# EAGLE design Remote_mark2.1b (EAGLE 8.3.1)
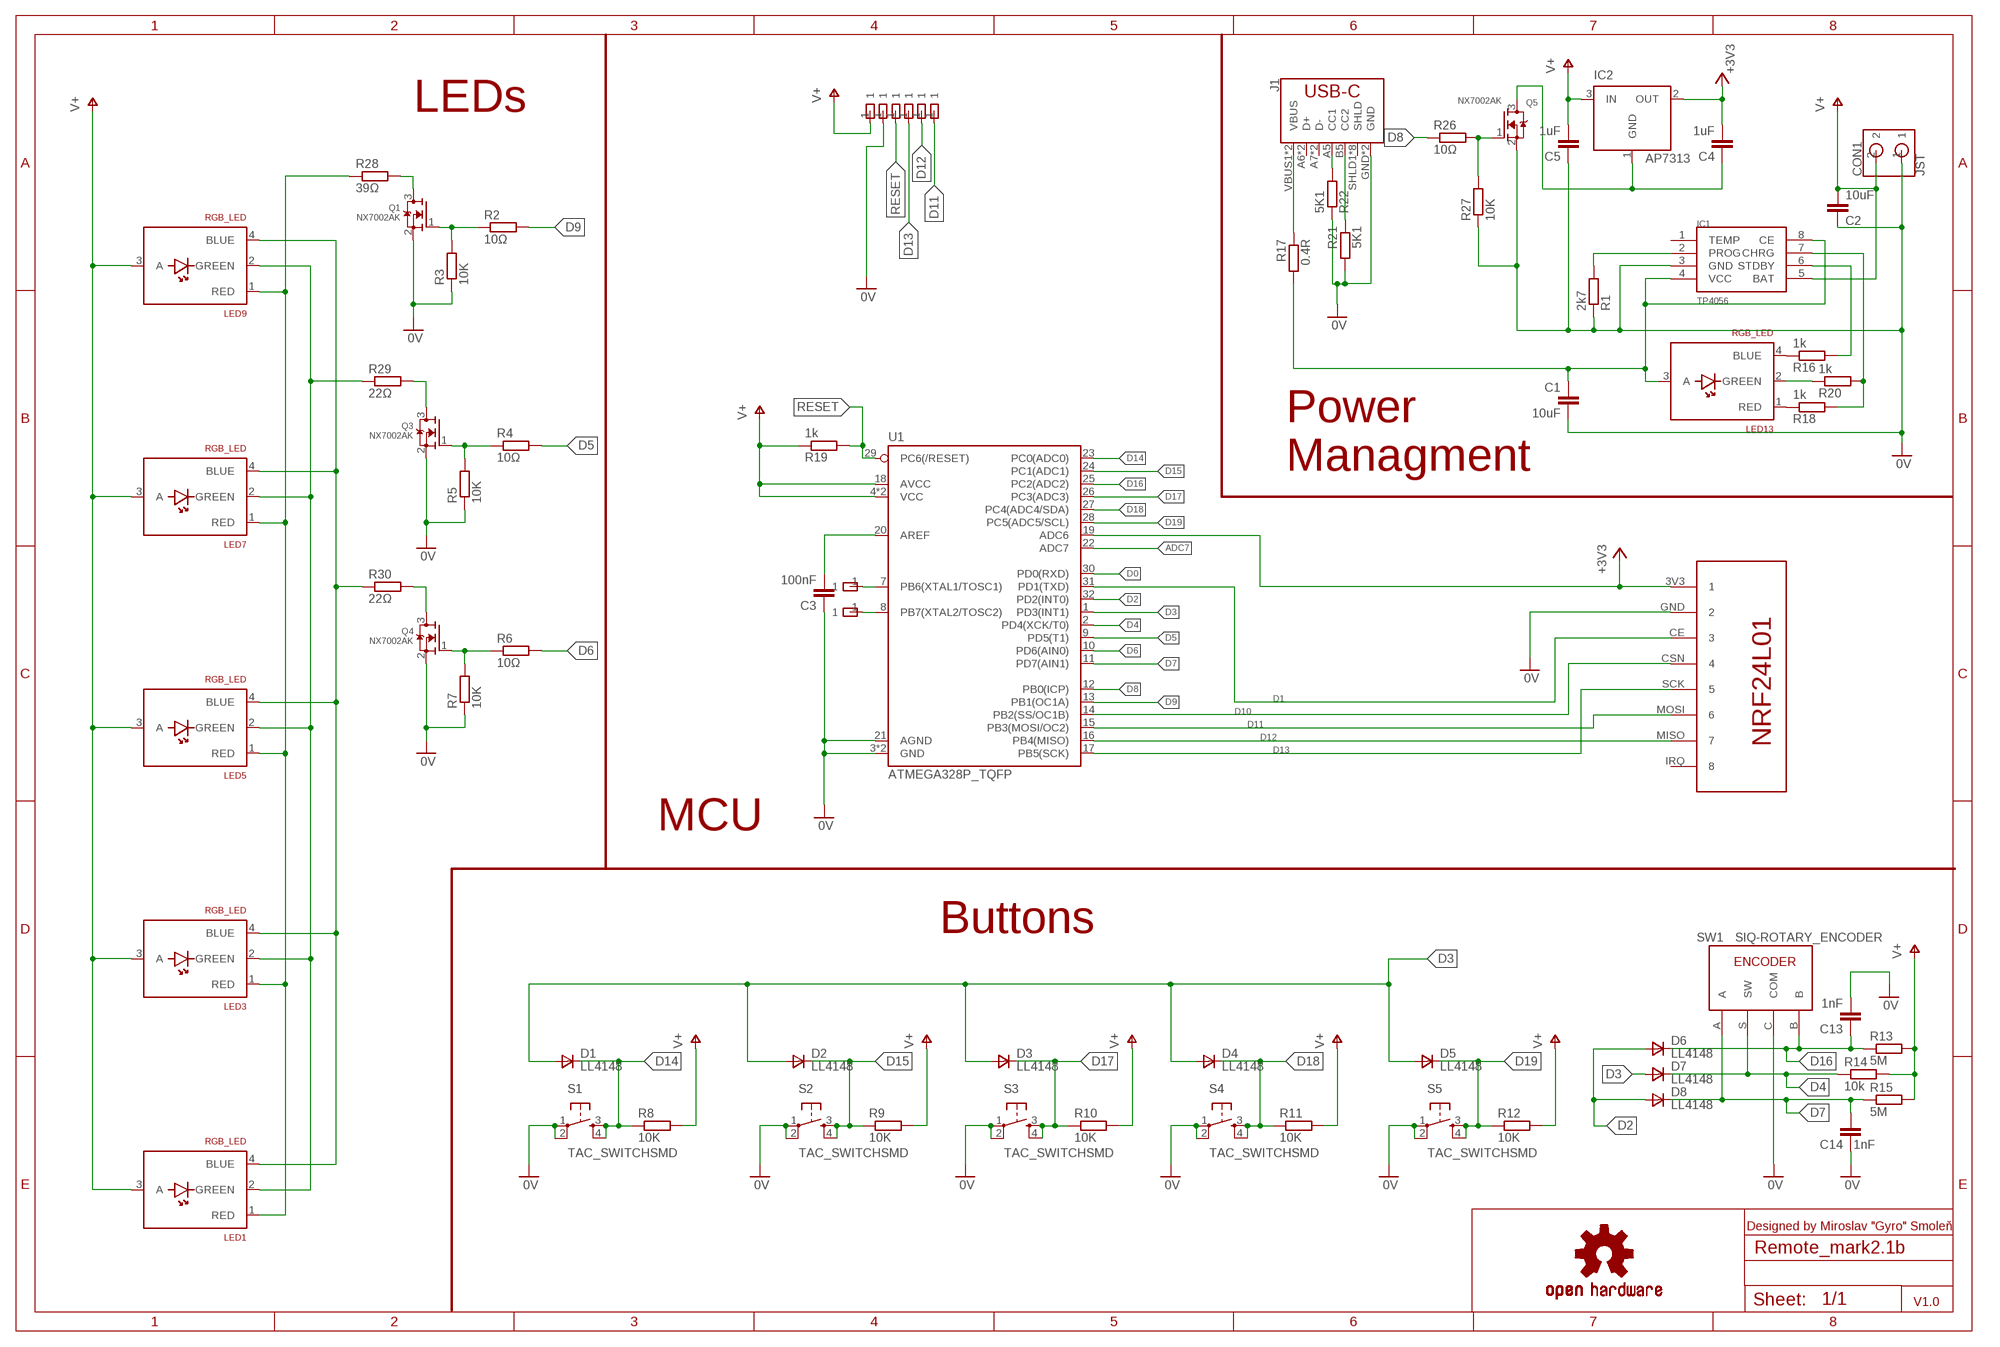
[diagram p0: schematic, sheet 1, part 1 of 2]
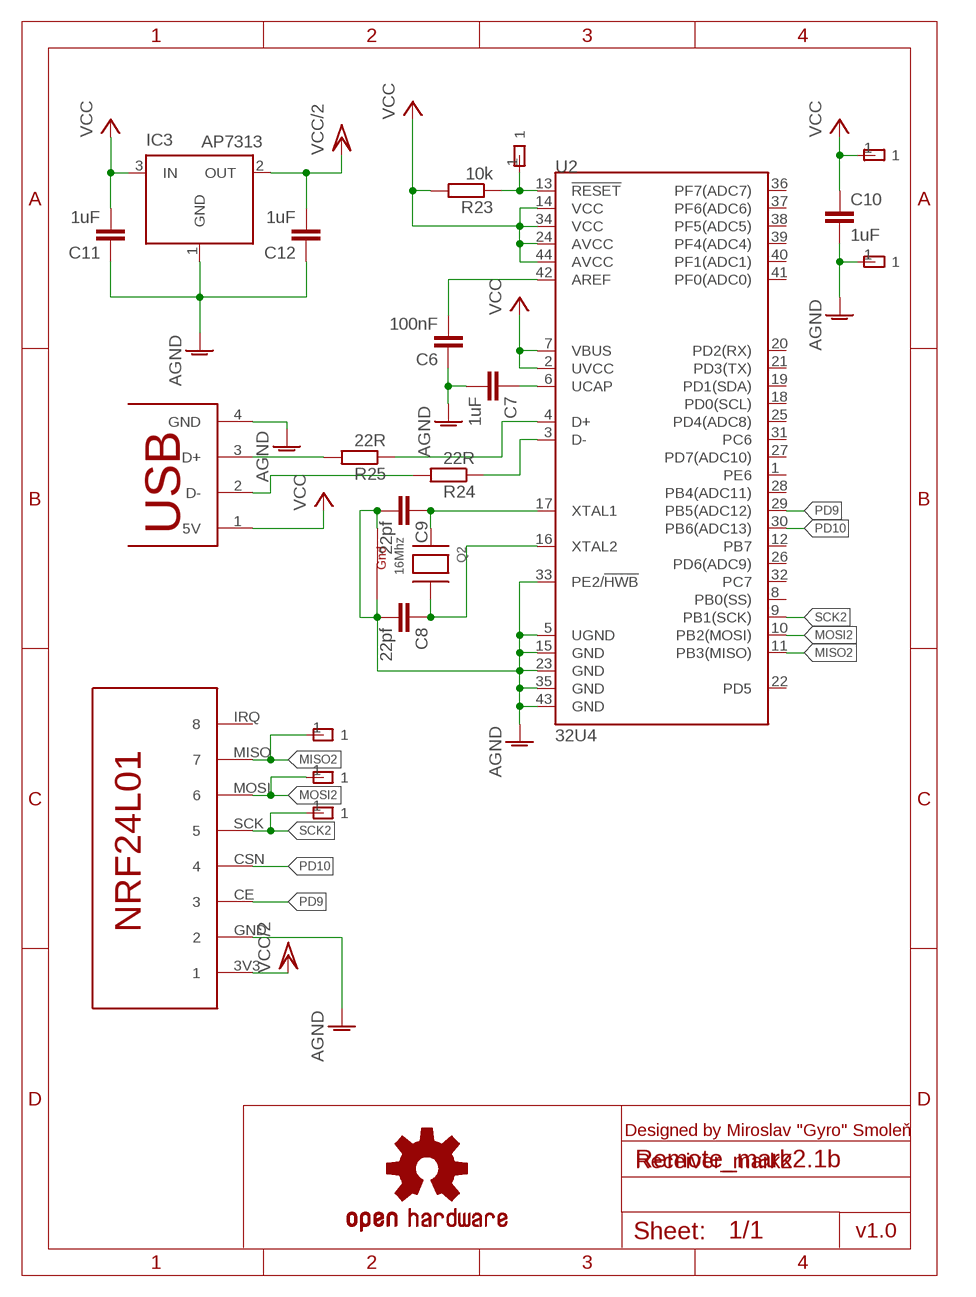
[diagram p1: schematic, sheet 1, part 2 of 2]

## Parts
C1  10uF  C-EUC0805  [C0805]
C2  10uF  C-EUC0805  [C0805]
C3  100nF  C-EUC0603  [C0603]
C4  1uF  C-EUC0603  [C0603]
C5  1uF  C-EUC0603  [C0603]
C6  100nF  C-EUC0603  [C0603]
C7  1uF  C-EUC0603  [C0603]
C8  22pf  C-EUC0603  [C0603]
C9  22pf  C-EUC0603  [C0603]
C10  1uF  C-EUC0603  [C0603]
C11  1uF  C-EUC0603  [C0603]
C12  1uF  C-EUC0603  [C0603]
C13  1nF  C-EUC0603  [C0603]
C14  1nF  C-EUC0603  [C0603]
CON1  JST  JST_PH2.0_BAT_CON  [JST_PH_2.0_2PIN_CONNECTOR]
D1  LL4148  DSOD323  [SOD323]
D2  LL4148  DSOD323  [SOD323]
D3  LL4148  DSOD323  [SOD323]
D4  LL4148  DSOD323  [SOD323]
D5  LL4148  DSOD323  [SOD323]
D6  LL4148  DSOD323  [SOD323]
D7  LL4148  DSOD323  [SOD323]
D8  LL4148  DSOD323  [SOD323]
IC1  TP4056  [SOP-8]
IC2  AP7313  AP7313_LINEAR_PWR_REG  [SOT23R]
IC3  AP7313  AP7313_LINEAR_PWR_REG  [SOT23R]
J1  USB_C16PIN  [USB-C-16P]
LED1  RGB_LED  [1.6X1.6_RGB_LED]
LED3  RGB_LED  [1.6X1.6_RGB_LED]
LED5  RGB_LED  [1.6X1.6_RGB_LED]
LED7  RGB_LED  [1.6X1.6_RGB_LED]
LED9  RGB_LED  [1.6X1.6_RGB_LED]
LED13  RGB_LED  [1.6X1.6_RGB_LED]
LOGO1  OSHW-LOGOS  [OSHW-LOGO-S]
LOGO2  OSHW-LOGOS  [OSHW-LOGO-S]
Q1  NX7002AK  MOSFET-NREFLOW  [SOT23]
Q2  16Mhz  XTAL-4-3225  [NX3225]
Q3  NX7002AK  MOSFET-NREFLOW  [SOT23]
Q4  NX7002AK  MOSFET-NREFLOW  [SOT23]
Q5  NX7002AK  MOSFET-NREFLOW  [SOT23]
R1  2k7  R-EU_R0603  [R0603]
R2  10Ω  R-EU_R0603  [R0603]
R3  10K  R-EU_R0603  [R0603]
R4  10Ω  R-EU_R0603  [R0603]
R5  10K  R-EU_R0603  [R0603]
R6  10Ω  R-EU_R0603  [R0603]
R7  10K  R-EU_R0603  [R0603]
R8  10K  R-EU_R0603  [R0603]
R9  10K  R-EU_R0603  [R0603]
R10  10K  R-EU_R0603  [R0603]
R11  10K  R-EU_R0603  [R0603]
R12  10K  R-EU_R0603  [R0603]
R13  5M  R-EU_R0603  [R0603]
R14  10k  R-EU_R0603  [R0603]
R15  5M  R-EU_R0603  [R0603]
R16  1k  R-EU_R0603  [R0603]
R17  0.4R  R-EU_R0805  [R0805]
R18  1k  R-EU_R0603  [R0603]
R19  1k  R-EU_R0603  [R0603]
R20  1k  R-EU_R0603  [R0603]
R21  5K1  R-EU_R0603  [R0603]
R22  5K1  R-EU_R0603  [R0603]
R23  10k  R-EU_R0603  [R0603]
R24  22R  R-EU_R0603  [R0603]
R25  22R  R-EU_R0603  [R0603]
R26  10Ω  R-EU_R0603  [R0603]
R27  10K  R-EU_R0603  [R0603]
R28  39Ω  R-EU_R0603  [R0603]
R29  22Ω  R-EU_R0603  [R0603]
R30  22Ω  R-EU_R0603  [R0603]
S1  TAC_SWITCHSMD  [TACTILE-SWITCH-SMD]
S2  TAC_SWITCHSMD  [TACTILE-SWITCH-SMD]
S3  TAC_SWITCHSMD  [TACTILE-SWITCH-SMD]
S4  TAC_SWITCHSMD  [TACTILE-SWITCH-SMD]
S5  TAC_SWITCHSMD  [TACTILE-SWITCH-SMD]
SW1  SIQ-ROTARY_ENCODER  [SIQ-02FVS3]
U1  ATMEGA328P_TQFP  [TQFP32-08]
U2  32U4  ATMEGA32U4TQFP-44  [TQFP44]
U$1  NRF24  [NRF24L01_SMT]
U$2  PAD_POGO_PIN  [POGO_PAD]
U$3  PAD_POGO_PIN  [POGO_PAD]
U$4  PAD_POGO_PIN  [POGO_PAD]
U$5  PAD_POGO_PIN  [POGO_PAD]
U$6  PAD_POGO_PIN  [POGO_PAD]
U$7  PAD_POGO_PIN  [POGO_PAD]
U$8  USB-A  [USB-A-SMT-MALE]
U$9  NRF24  [NRF24L01_SMT]
U$10  PAD_POGO_PIN  [POGO_PAD]
U$11  PAD_POGO_PIN  [POGO_PAD]
U$12  PAD_POGO_PIN  [POGO_PAD]
U$13  PAD_POGO_PIN  [POGO_PAD]
U$14  PAD_POGO_PIN  [POGO_PAD]
U$15  PAD_POGO_PIN  [POGO_PAD]
U$16  PAD_POGO_PIN  [POGO_PAD]
U$17  PAD_POGO_PIN  [POGO_PAD]

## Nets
0V: C1.2 C2.1 C3.1 C5.1 C13.2 C14.1 CON1.1 IC1.3(GND) J1.GND J1.GND2(GND) Q1.2(S) Q3.2(S) Q4.2(S) Q5.2(S) R1.1 R3.1 R5.1 R7.1 R21.2 R22.1 R27.1 S1.1 S1.2 S2.1 S2.2 S3.1 S3.2 S4.1 S4.2 S5.1 S5.2 SW1.C(COM) U1.3(GND) U1.5(GND) U1.21(AGND) U$1.GND U$3.1
+3V3: C4.2 IC2.2(OUT) U1.19(ADC6) U$1.3V3
ADC7: U1.22(ADC7)
AGND: C6.1 C7.2 C8.2 C9.2 C10.2 C11.1 C12.1 IC3.1(GND) Q2.2(G2) Q2.4(G1) U2.5(UGND) U2.15(GND) U2.23(GND) U2.33(PE2/!HWB) U2.35(GND) U2.43(GND) U$8.4(GND) U$9.GND U$17.1
D0: U1.30(PD0(RXD))
D1: U1.31(PD1(TXD)) U$1.CE
D2: D6.2(A) D8.2(A) U1.32(PD2(INT0))
D3: D1.2(A) D2.2(A) D3.2(A) D4.2(A) D5.2(A) D7.2(A) U1.1(PD3(INT1))
D4: D7.1(C) R14.1 SW1.S(SW) U1.2(PD4(XCK/T0))
D5: R4.2 U1.9(PD5(T1))
D6: R6.2 U1.10(PD6(AIN0))
D7: C14.2 D8.1(C) R15.1 SW1.A U1.11(PD7(AIN1))
D8: R26.1 U1.12(PB0(ICP))
D9: R2.2 U1.13(PB1(OC1A))
D10: U1.14(PB2(SS/OC1B)) U$1.CSN
D11: U1.15(PB3(MOSI/OC2)) U$1.MOSI U$7.1
D12: U1.16(PB4(MISO)) U$1.MISO U$6.1
D13: U1.17(PB5(SCK)) U$1.SCK U$5.1
D14: D1.1(C) R8.1 S1.3 S1.4 U1.23(PC0(ADC0))
D15: D2.1(C) R9.1 S2.3 S2.4 U1.24(PC1(ADC1))
D16: C13.1 D6.1(C) R13.1 SW1.B U1.25(PC2(ADC2))
D17: D3.1(C) R10.1 S3.3 S3.4 U1.26(PC3(ADC3))
D18: D4.1(C) R11.1 S4.3 S4.4 U1.27(PC4(ADC4/SDA))
D19: D5.1(C) R12.1 S5.3 S5.4 U1.28(PC5(ADC5/SCL))
MISO2: U2.11(PB3(MISO)) U$9.MISO U$12.1
MOSI2: U2.10(PB2(MOSI)) U$9.MOSI U$13.1
N$1: IC1.2(PROG) R1.2
N$2: LED1.1(RED) LED3.1(RED) LED5.1(RED) LED7.1(RED) LED9.1(RED) R28.1
N$3: C1.1 IC1.4(VCC) IC1.8(CE) LED13.3(A) R17.2
N$4: LED1.2(GREEN) LED3.2(GREEN) LED5.2(GREEN) LED7.2(GREEN) LED9.2(GREEN) R29.1
N$5: Q1.1(G) R2.1 R3.2
N$6: Q3.1(G) R4.1 R5.2
N$7: LED1.4(BLUE) LED3.4(BLUE) LED5.4(BLUE) LED7.4(BLUE) LED9.4(BLUE) R30.1
N$8: Q4.1(G) R6.1 R7.2
N$9: IC1.6(STDBY) R16.2
N$10: IC1.7(CHRG) R18.2 R20.2
N$11: LED13.4(BLUE) R16.1
N$12: LED13.1(RED) R18.1
N$13: C9.1 Q2.1(X1) U2.17(XTAL1)
N$14: C3.2 U1.20(AREF)
N$16: LED13.2(GREEN) R20.1
N$17: J1.B5(CC2) R21.1
N$18: J1.A5(CC1) R22.2
N$19: C8.1 Q2.3(X2) U2.16(XTAL2)
N$20: C6.2 U2.42(AREF)
N$21: J1.VBUS1(VBUS) J1.VBUS2(VBUS) R17.1
N$22: U1.7(PB6(XTAL1/TOSC1)) U$10.1
N$23: C7.1 U2.6(UCAP)
N$24: R23.1 U2.13(!RESET) U$15.1
N$25: U1.8(PB7(XTAL2/TOSC2)) U$11.1
N$26: R24.1 U2.3(D-)
N$27: R25.1 U2.4(D+)
N$28: R25.2 U$8.3(D+)
N$29: R24.2 U$8.2(D-)
N$30: Q5.1(G) R26.2 R27.2
N$31: C4.1 IC2.1(GND) Q5.3(D)
N$32: Q1.3(D) R28.2
N$33: Q3.3(D) R29.2
N$34: Q4.3(D) R30.2
PD9: U2.29(PB5(ADC12)) U$9.CE
PD10: U2.30(PB6(ADC13)) U$9.CSN
RESET: R19.2 U1.29(PC6(/RESET)) U$4.1
SCK2: U2.9(PB1(SCK)) U$9.SCK U$14.1
V+: C2.2 C5.2 CON1.2 IC1.5(BAT) IC2.3(IN) LED1.3(A) LED3.3(A) LED5.3(A) LED7.3(A) LED9.3(A) R8.2 R9.2 R10.2 R11.2 R12.2 R13.2 R14.2 R15.2 R19.1 U1.4(VCC) U1.6(VCC) U1.18(AVCC) U$2.1
VCC: C10.1 C11.2 IC3.3(IN) R23.2 U2.2(UVCC) U2.7(VBUS) U2.14(VCC) U2.24(AVCC) U2.34(VCC) U2.44(AVCC) U$8.1(5V) U$16.1
VCC/2: C12.2 IC3.2(OUT) U$9.3V3
Unconnected: IC1.1(TEMP) J1.A6(D+) J1.A7(D-) J1.B6(D+) J1.B7(D-) J1.SHLD1(SHLD) J1.SHLD2(SHLD) J1.SHLD3(SHLD) J1.SHLD4(SHLD) J1.SHLD5(SHLD) J1.SHLD6(SHLD) J1.SHLD7(SHLD) J1.SHLD8(SHLD) U2.1(PE6) U2.8(PB0(SS)) U2.12(PB7) U2.18(PD0(SCL)) U2.19(PD1(SDA)) U2.20(PD2(RX)) U2.21(PD3(TX)) U2.22(PD5) U2.25(PD4(ADC8)) U2.26(PD6(ADC9)) U2.27(PD7(ADC10)) U2.28(PB4(ADC11)) U2.31(PC6) U2.32(PC7) U2.36(PF7(ADC7)) U2.37(PF6(ADC6)) U2.38(PF5(ADC5)) U2.39(PF4(ADC4)) U2.40(PF1(ADC1)) U2.41(PF0(ADC0)) U$1.IRQ U$9.IRQ

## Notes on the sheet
- LEDs
- Power
  Managment
- MCU
- Buttons
- Designed by Miroslav "Gyro" Smoleň | Designed by Miroslav "Gyro" Smoleň
- Receiver_mark2
- V1.0 | v1.0

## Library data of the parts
C1-C14 = rcl:C-EU: CAPACITOR, European symbol
CON1 = Gyro_library:JST_PH2.0_BAT_CON
D1-D8 = zetex:D: DIODE; MPN: CDSOD323-T05C; OC_FARNELL: 1824860; OC_NEWARK: 79R6078
IC1 = TP4056:TP4056
IC2 IC3 = Gyro_library:AP7313_LINEAR_PWR_REG: 1.2V Voltage Reference 50ppm/°C, SOT23, 3-Terminal Source: Data sheet; MF: MAXIM; MPN: MAX6520EUR-T; OC_FARNELL: unknown; OC_NEWARK: 02J4586
J1 = SparkFun-Connectors:USB_C: USB Type C 16Pin Connector Super Speed pins not available on the 16-pin purely SMD connector so this part is best for USB 2.0 implementations. D1 and D2 are tied together enabling D+/- no matter which way the cable is plugged into the connector. The two channel configuration pins (CC1/2) are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; PROD_ID: CONN-14122
LED1 LED3 LED5 LED7 LED9 LED13 = Gyro_library:RGB_LED
LOGO1 LOGO2 = SparkFun-Aesthetics:OSHW-LOGO: Open-Source Hardware (OSHW) Logo
Q1 Q3-Q5 = adafruit:MOSFET-N: N-Channel Mosfet 2N7002E - 60V 260mA SOT23 [Digikey: 2N7002ET1GOSTR-ND] - REEL BSH103 - 30V 850mA SOT23 [Digikey: 568-5013-1-ND]
Q2 = adafruit:XTAL-4: Classic 4-pin 3.2 x 2.5mm crystal
R1-R30 = rcl:R-EU_: RESISTOR, European symbol
S1-S5 = SparkFun-Retired:TAC_SWITCH: Momentary Switch Button commonly used for reset or general input. Spark Fun Electronics SKU : COM-00097 SMT- SWCH-08247; PROD_ID: SWCH-08247
SW1 = Gyro_library:SIQ-ROTARY_ENCODER
U1 = SparkFun-IC-Microcontroller:ATMEGA328P_TQFP: Popular 328P in QFP Storefront component: ATmega328 - TQFP (COM-13448) Datasheet SparkFun Products SparkFun RedBoard - Programmed with Arduino (DEV-12757) Arduino Pro Mini 328 - 5V/16MHz (DEV-11113) Arduino Pro Mini 328 - 3.3V/8MHz (DEV-11114) SparkFun OpenLog (DEV-13712) SparkFun MicroView - OLED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; PROD_ID: IC-09069
U2 = SparkFun-IC-Microcontroller:ATMEGA32U4: Atmel MCU, 32KByte Atmel 44-pin 8-bit Microcontroller with 32KBytes of ISP Flash and USB Controller Datasheet SparkFun Products LilyPad Arduino USB - ATmega32U4 Board (DEV-12049) Pro Micro - 5V/16MHz (DEV-12640) Pro Micro - 3.3V/8MHz (DEV-12587) Fio v3 - ATmega32U4 (DEV-11520) Qduino Mini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; PROD_ID: IC-11161
U$1 U$9 = Gyro_library:NRF24: SMD version of NRF24L01 wireless transceiver module. Made by Gyro: https://www.youtube.com/c/gyro1
U$2-U$7 U$10-U$17 = Gyro_library:PAD_POGO_PIN
U$8 = Gyro_library:USB-A

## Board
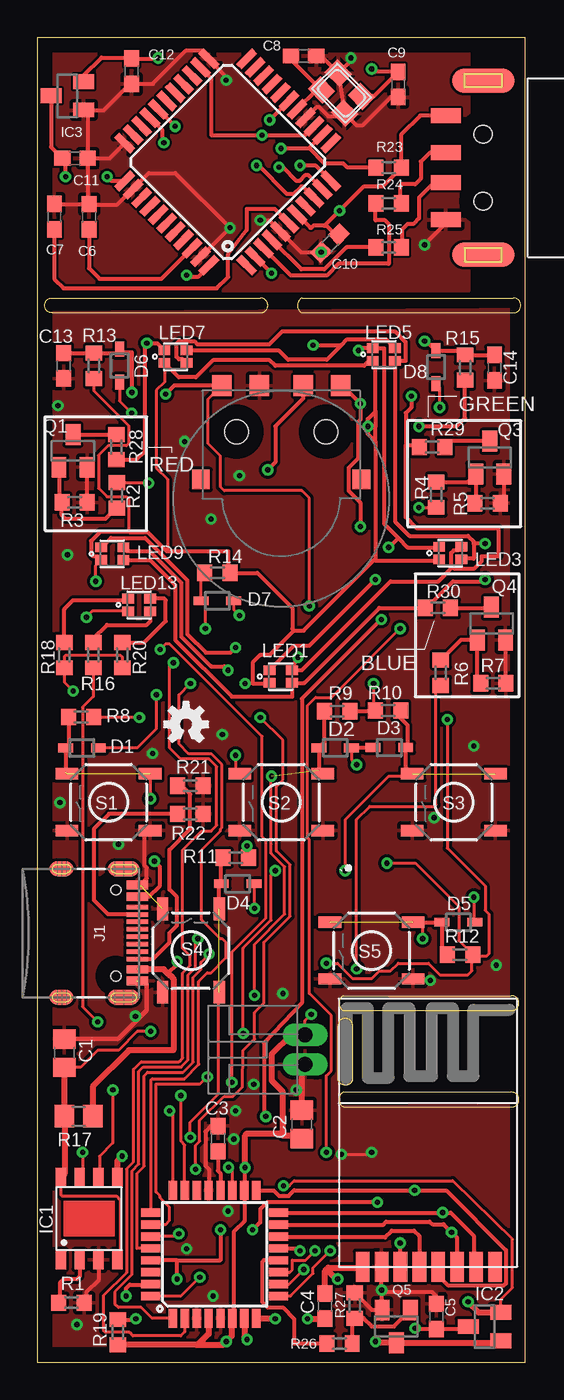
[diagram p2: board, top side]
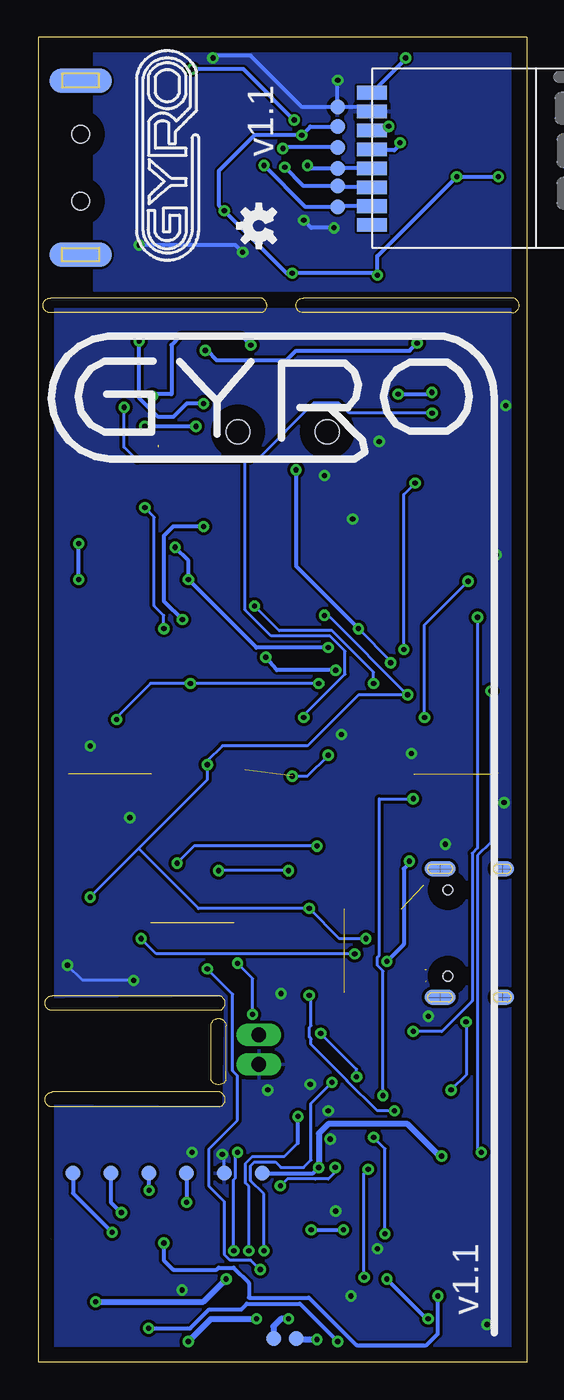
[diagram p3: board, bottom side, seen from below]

Size 32.8 x 89 mm. Coordinates in mm from the lower left corner, seen from the top.
Outline: 0,0 32.8,0 32.8,89 0,89 0,0
Copper layers (1*16): Top 0.035mm / dielectric 1.5mm / Bottom 0.035mm
Design rules "default": minimum track width 6mil, minimum drill 0.35mm, track to track 6mil, track to pad 6mil, pad to pad 6mil, via to via 6mil, smd to smd 6mil, copper to edge 40mil, drill to drill 6mil, minimum pad ring 10mil, minimum via ring 8mil, stop-mask expansion 4mil, vias tented up to drill 0mil, thermal gap 10mil
Milling: 20 lines

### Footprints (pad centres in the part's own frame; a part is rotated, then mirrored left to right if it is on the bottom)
C0805 = smd 1.3 x 1.5: 1 -0.95,0; 2 0.95,0
C0603 = smd 1.1 x 1: 1 -0.85,0; 2 0.85,0
JST_PH_2.0_2PIN_CONNECTOR = drill 1 long: 1 -1,0; 2 1,0
SOD323 = smd 1 x 0.6: 1 -1.1,0; 2 1.1,0
SOP-8 = smd 1.3 x 0.7: 1 -2.75,1.905; 2 -2.75,0.635; 3 -2.75,-0.635; 4 -2.75,-1.905; 5 2.75,-1.905; 6 2.75,-0.635; 7 2.75,0.635; 8 2.75,1.905
SOT23R = smd 1 x 1.4: 1 -0.95,-1.1; 2 0.95,-1.1; 3 0,1.1
USB-C-16P = smd 0.3 x 1.45: A5 -1.25,0; A6 -0.25,0; A7 0.25,0; A8 1.25,0; B5 1.75,0; B6 0.75,0; B7 -0.75,0; B8 -1.75,0 | smd 0.6 x 1.45: GND -3.225,0; GND2 3.225,0 | smd 1 x 2.1: SHLD1 -4.32,-0.915; SHLD2 4.32,-0.915 | smd 1 x 2.1 bottom: SHLD3 -4.32,-0.915; SHLD4 4.32,-0.915 | smd 1 x 1.6: SHLD5 -4.32,-5.095; SHLD8 4.32,-5.095 | smd 1 x 1.6 bottom: SHLD6 -4.32,-5.095; SHLD7 4.32,-5.095 | smd 0.55 x 1.45: VBUS1 -2.45,0; VBUS2 2.45,0 | hole 0.65: -2.89,-1.445; 2.89,-1.445
1.6X1.6_RGB_LED = smd 0.8 x 0.65: 1 -0.75,0.425; 2 0.75,0.425; 3 -0.75,-0.425; 4 0.75,-0.425
SOT23 = smd 1 x 1.4: 1 -0.95,-1.1; 2 0.95,-1.1; 3 0,1.1
NX3225 = smd 1.4 x 1.2: 1 -1.1,-0.8; 2 1.1,-0.8; 3 1.1,0.8; 4 -1.1,0.8
R0603 = smd 1 x 1.1: 1 -0.85,0; 2 0.85,0
R0805 = smd 1.3 x 1.5: 1 -0.95,0; 2 0.95,0
TACTILE-SWITCH-SMD = smd 1.524 x 0.762: 1 -2.794,1.905; 2 2.794,1.905; 3 -2.794,-1.905; 4 2.794,-1.905
SIQ-02FVS3 = smd 1.3 x 1.4: A -4,-7.6; B 4,-7.6; C 1.475,-7.6; S -1.475,-7.6 | smd 1.2 x 1.3: P$5 5.4,-1.3; P$6 -5.4,-1.3 | hole 1.6: -3,-4.5; 3,-4.5
TQFP32-08 = smd 1.27 x 0.559: 1 -4.293,2.8; 2 -4.293,2; 3 -4.293,1.2; 4 -4.293,0.4; 5 -4.293,-0.4; 6 -4.293,-1.2; 7 -4.293,-2; 8 -4.293,-2.8; 17 4.293,-2.8; 18 4.293,-2; 19 4.293,-1.2; 20 4.293,-0.4; 21 4.293,0.4; 22 4.293,1.2; 23 4.293,2; 24 4.293,2.8 | smd 0.559 x 1.27: 9 -2.8,-4.293; 10 -2,-4.293; 11 -1.2,-4.293; 12 -0.4,-4.293; 13 0.4,-4.293; 14 1.2,-4.293; 15 2,-4.293; 16 2.8,-4.293; 25 2.8,4.293; 26 2,4.293; 27 1.2,4.293; 28 0.4,4.293; 29 -0.4,4.293; 30 -1.2,4.293; 31 -2,4.293; 32 -2.8,4.293
TQFP44 = smd 1.5 x 0.5: 1 -5.8,4; 2 -5.8,3.2; 3 -5.8,2.4; 4 -5.8,1.6; 5 -5.8,0.8; 6 -5.8,0; 7 -5.8,-0.8; 8 -5.8,-1.6; 9 -5.8,-2.4; 10 -5.8,-3.2; 11 -5.8,-4; 23 5.8,-4; 24 5.8,-3.2; 25 5.8,-2.4; 26 5.8,-1.6; 27 5.8,-0.8; 28 5.8,0; 29 5.8,0.8; 30 5.8,1.6; 31 5.8,2.4; 32 5.8,3.2; 33 5.8,4 | smd 0.5 x 1.5: 12 -4,-5.8; 13 -3.2,-5.8; 14 -2.4,-5.8; 15 -1.6,-5.8; 16 -0.8,-5.8; 17 0,-5.8; 18 0.8,-5.8; 19 1.6,-5.8; 20 2.4,-5.8; 21 3.2,-5.8; 22 4,-5.8; 34 4,5.8; 35 3.2,5.8; 36 2.4,5.8; 37 1.6,5.8; 38 0.8,5.8; 39 0,5.8; 40 -0.8,5.8; 41 -1.6,5.8; 42 -2.4,5.8; 43 -3.2,5.8; 44 -4,5.8
NRF24L01_SMT = smd 2 x 0.914: 3V3 -9,4.4; CE -9,1.86; CSN -9,0.59; GND -9,3.13; IRQ -9,-4.49; MISO -9,-3.22; MOSI -9,-1.95; SCK -9,-0.68
POGO_PAD = smd 1 x 1: 1 0,0
USB-A-SMT-MALE = smd 1 x 2: 1 3.5,2.5; 2 1,2.5; 3 -1,2.5; 4 -3.5,2.5 | smd 1.651 x 4.191 bottom: P$1 -5.842,0; P$2 5.842,0 | smd 1.651 x 4.191: P$3 5.842,0; P$5 -5.842,0 | hole 1.2: 2.25,0; -2.25,0

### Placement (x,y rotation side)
C1  1.83,20.76 90 top
C2  17.78,15.98 270 top
C3  12.15,15.02 270 top
C4  19.35,3.78 90 top
C5  26.82,3.08 270 top
C6  3.48,76.94 270 top
C7  1.16,76.94 90 top
C8  17.91,87.74 0 top
C9  24.26,85.83 270 top
C10  19.68,75.16 225 top
C11  2.54,80.87 180 top
C12  6.35,86.71 90 top
C13  1.78,66.93 270 top
C14  30.73,66.8 90 top
CON1  18,21 90 top
D1  3.01,41.26 0 top
D2  20.03,41.27 0 top
D3  23.66,41.29 180 top
D4  13.47,32.15 0 top
D5  28.3,29.56 0 top
D6  5.53,66.94 270 top
D7  12.1,51.15 0 top
D8  26.8,66.84 270 top
IC1  3.49,9.65 90 top
IC2  30.06,2.4 90 top
IC3  2.03,85.06 90 top
J1  6.73,28.83 270 top
LED1  16.36,46.06 0 top
LED3  27.76,54.35 0 top
LED5  23.29,67.69 0 top
LED7  9.3,67.55 0 top
LED9  5.04,54.31 0 top
LED13  6.85,50.87 0 top
LOGO1  10,42.85 0 top
LOGO2  18,76.33 90 bottom
Q1  2.41,61.21 0 top
Q2  20.45,85.24 135 top
Q3  30.41,60.76 0 top
Q4  30.52,49.62 0 top
Q5  24.13,2.41 180 top
R1  2.3,4 180 top
R2  5.34,58.23 90 top
R3  2.52,57.75 180 top
R4  26.81,58.27 270 top
R5  30.27,57.7 180 top
R6  27.12,46.32 270 top
R7  30.65,45.6 180 top
R8  2.95,43.34 0 top
R9  20.16,43.73 0 top
R10  23.59,43.78 180 top
R11  13.35,33.89 0 top
R12  28.41,27.39 0 top
R13  3.81,66.93 270 top
R14  12.11,53.02 0 top
R15  28.74,66.81 270 top
R16  3.77,47.5 270 top
R17  2.79,16.53 180 top
R18  1.82,47.5 270 top
R19  5.43,2.02 90 top
R20  5.71,47.5 270 top
R21  10.29,38.73 0 top
R22  10.29,36.83 180 top
R23  23.62,80.24 0 top
R24  23.62,77.82 0 top
R25  23.62,74.89 0 top
R26  20.32,1.27 0 top
R27  21.34,3.81 270 top
R28  5.33,61.47 90 top
R29  26.54,61.47 0 top
R30  26.92,50.67 0 top
S1  4.8,37.62 180 top
S2  16.4,37.62 180 top
S3  28,37.62 180 top
S4  10.33,27.65 90 top
S5  22.47,27.65 180 top
SW1  16.4,58 180 top
U1  11.92,7.25 90 top
U2  12.81,80.62 135 top
U$1  26.27,15.42 90 top
U$2  17.78,12.7 270 bottom
U$3  20.32,12.7 270 bottom
U$4  22.86,12.7 270 bottom
U$5  25.4,12.7 270 bottom
U$6  27.94,12.7 270 bottom
U$7  30.48,12.7 270 bottom
U$8  29.97,80.24 90 top
U$9  1.4,80.87 0 bottom
U$10  15.5,1.6 0 bottom
U$11  17,1.6 0 bottom
U$12  12.7,77.6 0 bottom
U$13  12.7,79 0 bottom
U$14  12.7,80.18 0 bottom
U$15  12.7,81.6 0 bottom
U$16  12.7,83 0 bottom
U$17  12.7,84.3 0 bottom

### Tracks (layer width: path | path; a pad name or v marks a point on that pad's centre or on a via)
0V  (via drill 0.35)  (2 unrouted)
  Top 0.203: S5.1 26.32,25.75 v26.42,25.65 | v20.45,13.97 22.35,13.97 v22.48,14.1
  Top 0.254: R27.1 22.48,3.51 Q5.2 23.14,3.55 23.14,4.71 | 23.14,4.71 U$1.GND | R3.1 3.37,60.11 Q1.2 | Q3.2 31.36,57.95 R5.1 | Q4.2 31.47,45.63 R7.1 | IC1.3 4.12,5.52 3.3,4.7 3.3,4.15 R1.1 | J1.GND 6.91,32.05 7.37,32.51 7.37,33.23 7.22,33.38 7.22,35.33 S1.1 | C3.1 11.68,15.87 11.3,15.49 11.3,13.21 11.56,12.95 11.56,11.58 U1.21 | C5.1 26.82,4.43 26.54,4.7 23.15,4.7 23.14,4.71
  Top 0.305: C1.2 5.46,21.71 7.37,23.62 7.37,25.4 7.24,25.53 6.81,25.53 6.78,25.56
  Top 0.406: C2.1 17.78,19.78 CON1.1
  Bottom 0.203: v26.42,25.65 29.84,25.65 v30.86,26.67 | U$3.1 20.32,13.84 v20.45,13.97
  other vias: 11.68,56.64 9.91,61.85 13.59,59.56 1.4,64.26 5.46,34.8 7.75,40.89 12.45,42.16 29.34,41.4 11.81,4.45 2.67,2.54 23.15,4.85 13.21,14.99 16.51,24.77 17.4,18.29 26.67,36.58 1.52,37.59 6.6,23.24 12.83,10.16 2.03,54.23 10.03,7.62 13.34,16.89 14.55,18.66
  pour Top (isolate 0.2): 0,-0.13 33.53,-0.13 34.16,17.27 20.32,17.14 20.19,24.64 34.04,24.51 34.67,70.74 0,70.48
  pour Bottom (isolate 0.2): -0.51,-0.64 33.91,-0.64 33.53,17.27 20.32,17.14 20.19,24.64 34.67,24.51 33.91,70.74 -0.51,70.74
+3V3  (via drill 0.35)  (1 unrouted)
  Top 0.203: IC2.2 31.16,4.24 31.94,5.01 31.94,8.25 | U1.19 13.12,12.83 v12.86,13.09 | v16.55,11.85 16.93,11.85 17.27,12.19 27.92,12.19 31.95,8.26
  Top 0.406: C4.2 19.35,6.14 19.45,6.24 | 19.45,6.24 19.56,6.35 21.8,6.35 U$1.3V3 | IC2.2 29.67,3.35 v28.96,4.06 | v20.19,5.59 20.1,5.59 19.45,6.24
  Bottom 0.203: v12.86,13.09 12.86,12.79 13.34,12.32 14.19,12.32 | 14.19,12.32 | v16.55,11.85 16.08,12.32 14.19,12.32
  Bottom 0.406: v28.96,4.06 21.72,4.06 v20.19,5.59
AGND  (via drill 0.35)
  Top 0.254: C10.2 17.74,74.56 U2.5 15.58,76.71 v14.99,76.71 | Q2.2 Q2.4 | C9.2 23.76,84.97 21.84,83.06 21.5,83.06 Q2.4 | C8.2 19.08,87.74 Q2.2 | C11.1 3.39,83.86 3.22,84.03 | 3.22,84.03 IC3.1 | 3.22,84.03 3.27,84.07 4.45,84.07 6.24,85.86 C12.1 7.76,85.86 10.01,88.11 11.05,88.11 11.56,87.63 11.53,87.53 12.7,86.36 v12.7,86.11 | C11.1 3.39,77.88 C6.1 | C7.2 C6.1 | C6.1 3.54,77.72 5.33,77.72 6.39,78.78 U2.35 6.44,78.83 7.49,79.88 9.27,79.88 v12.95,76.2 11.01,74.25 U2.43 | C11.1 4.86,80.87 U2.33 | U$8.4 27.47,76.49 v26.04,75.06 | U2.15 18.06,83.59 18.8,84.33 18.92,84.33 19.56,83.69 20.47,83.69 Q2.4 | v21.08,87.61 21.08,87.43 Q2.2
  Bottom 0.254: U$17.1 10.7,84.3 U$9.GND | U$17.1 v12.7,86.11 | v26.04,75.06 19.59,75.06 C10.2 | v12.95,76.2 14.48,76.2 v14.99,76.71 | U$17.1 15.09,84.3 18.54,87.76 20.93,87.76 v21.08,87.61
  other vias: 19.08,74.56
  pour Top: 0,72 29,72 29,89 0,89.13
  pour Bottom: 0,72 29,72 29,89 0,89.13
D1  (via drill 0.35)
  Top 0.254: U$1.CE 24.41,7.97 v24.38,8 | v5.97,4.45 5.97,4.95 6.22,5.21 7.58,5.21 U1.31
  Bottom 0.254: v24.38,8 24.38,6.86 23.75,6.22 20.83,6.22 20.7,6.35 19.68,6.35 18.67,5.33 18.67,4.34 14.63,4.34 11.43,1.14 6.73,1.14 5.97,1.91 v5.97,4.45
D2  (via drill 0.35)
  Top 0.203: D6.2 5.53,64.57 v6.35,63.75 | v27.05,64.14 27.05,65.49 D8.2 | U1.32 9.66,4.45 v10.92,5.71 | v10.64,12.95 10.64,14.58 10.92,14.85 10.92,16.26 12.57,17.86 13.16,17.86 13.79,18.49 13.84,20.95 14.61,21.72 14.61,23.5 15.24,24.13 15.24,28.21 16.99,29.96 16.99,33.43 16.08,34.34 16.08,38.68 16.51,39.12 16.51,41.78 v14.99,43.31
  Bottom 0.203: v6.35,63.75 11.94,63.75 12.61,64.42 14.32,64.42 18.03,60.71 18.48,60.71 18.61,60.58 18.93,60.58 | 18.93,60.58 26.16,60.58 27.05,61.47 v27.05,64.14 | v10.92,5.71 10.92,12.68 v10.64,12.95 | v14.99,43.31 14.99,43.43 12.2,46.22 12.2,47.76 13.23,48.79 17.18,48.79 18.92,50.54 18.92,60.57 18.93,60.58
D3  (via drill 0.35)
  Top 0.203: U1.1 7.71,2.96 6.99,3.68 5.46,3.68 5.21,3.94 5.21,4.73 6.36,5.88 6.36,12.84 6.83,13.31 6.83,19.54 7.13,19.84 9.67,19.84 10.13,20.3 10.13,26.02 10.64,26.52 10.64,28.3 v10.79,28.45 | v14.61,30.48 14.61,32.11 D4.2 | D7.2 13.2,50.55 v13.59,50.16 | v8,44.83 8,42.55 6.73,41.27 4.13,41.27 D1.2 | D2.2 21.13,40.47 v21.46,40.13 | v29.34,31.24 29.34,29.62 D5.2
  Top 0.254: D2.2 22.55,41.27 D3.2
  Bottom 0.203: v10.79,28.45 12.57,28.45 v14.61,30.48 22.05,30.48 26.07,34.5 | v13.59,50.16 13.34,50.16 v8,44.83 11.3,44.83 14.73,41.4 20.45,41.4 21.46,40.39 v21.46,40.13 21.46,39.12 26.07,34.5 | 26.07,34.5 v29.34,31.24
D4  (via drill 0.35)
  Top 0.203: U1.2 9.92,2.05 9.65,1.78 6.42,1.78 6.2,2 4.6,2 4.45,2.16 4.45,4.47 6,6.03 6,12.98 6.48,13.46 6.48,19.68 6.99,20.19 9.53,20.19 9.78,20.45 9.78,26.16 10.29,26.67 10.29,27.3 9.78,27.81 9.78,34.42 11.05,35.69 11.68,35.69 12.06,36.07 12.06,40.01 11.56,40.51 9.65,40.51 8.89,41.27 8.89,46.74 v9.14,46.99 | v11.3,49.28 11.3,50.85 D7.1 11,52.77 R14.1
  Top 0.254: SW1.S 17.88,64.74 16,62.87 16,60.45 v15.49,59.94
  Bottom 0.203: v9.14,46.99 9.14,47.12 v11.3,49.28
  Bottom 0.254: v15.49,59.94 15.49,53.47 v11.3,49.28
D5  (via drill 0.35)
  Top 0.203: v19.68,7.49 18.54,6.35 18.54,5.96 17.03,4.45 U1.9 | v19.43,14.1 19.43,19.25 19.76,19.58 19.76,23.29 18.29,24.77 18.29,35.12 18.18,35.23 18.18,44.12 18.71,44.66 19.76,44.66 v24.38,49.28 | v25.65,57.4 26.79,57.4 R4.2
  Bottom 0.203: v19.68,7.49 19.68,12.27 19.57,12.39 19.57,13.96 v19.43,14.1 | v24.38,49.28 24.38,50.16 25.02,50.8 25.02,56.77 v25.65,57.4
D6  (via drill 0.35)
  Top 0.203: U1.10 16.93,5.25 v17.91,6.22 | v21.46,26.42 21.46,36.45 22.35,37.34 26.67,37.34 26.8,37.47 26.8,45.14 R6.2
  Bottom 0.203: v17.91,6.22 18.55,6.86 19.95,6.86 20.32,7.23 20.32,10.79 21.34,11.81 21.34,14.35 19.43,16.26 19.43,19.25 19.76,19.58 19.76,24.71 v21.46,26.42
D7  (via drill 0.35)
  Top 0.203: U1.11 16.97,6.05 17.14,6.22 17.14,6.86 18.03,6.86 v18.67,7.49
  Top 0.254: C14.2 30.72,67.66 R15.1 28.47,67.94 D8.1 26.16,68.58 v26.04,68.58 | SW1.A 20.51,65.6 v21.72,64.39 21.72,63.29 21.57,63.14 21.57,60.71 20.92,60.07 20.92,58.53 21.72,57.74 v21.72,56.13 | v23.13,49.89 23.09,49.89 17.78,44.58 17.78,24.13 15.24,21.46 15.24,16.76 v15.37,16.51
  Bottom 0.203: 15.37,14.73 16.28,13.82 18.43,13.82 18.9,13.36 18.9,12.04 18.67,11.82 v18.67,7.49
  Bottom 0.254: v21.72,64.39 22.86,64.39 23.75,63.5 24.77,63.5 26.04,64.77 v26.04,68.58 | v21.72,56.13 23.75,56.13 24.38,55.5 24.38,51.14 v23.13,49.89 | 15.37,14.73 v15.37,16.51
D8
  Top 0.254: U1.12 15.23,6.85 15.11,6.73 15.11,4.06 15.49,3.68 16.51,3.68 17.27,2.92 17.27,1.27 R26.1
D9  (via drill 0.35)
  Top 0.203: v13.08,18.8 13.08,27.56 15.37,29.84 15.37,35.05 15.11,35.31 15.11,42.04 8.89,48.26 8.64,48.26 v8.26,47.88 | v7.49,59.05 5.37,59.05 R2.2
  Top 0.254: U1.13 17.5,7.65 v17.65,7.49
  Bottom 0.203: v17.65,7.49 17.65,11.3 18.54,12.19 18.54,13.21 18.29,13.46 16.89,13.46 16.51,13.08 14.99,13.08 14.48,13.59 14.48,17.4 v13.08,18.8 | v8.26,47.88 8.26,58.29 v7.49,59.05
D10
  Top 0.254: U1.14 16.28,8.38 23.37,8.38 23.83,8.84 25.32,8.84 25.68,8.48 U$1.CSN
D11  (via drill 0.35)
  Top 0.254: U$1.MOSI 28.19,6.45 28.19,8.38 v27.85,8.72 27.3,9.27 26.54,9.27 26.36,9.45 23.45,9.45 23.25,9.25 U1.15
  Bottom 0.254: U$7.1 30.48,11.35 v27.85,8.72
D12  (via drill 0.35)
  Top 0.254: U1.16 v27.24,10.05 27.8,10.05 29.34,8.51 29.34,6.57 U$1.MISO
  Bottom 0.254: U$6.1 27.94,10.75 v27.24,10.05
D13  (via drill 0.35)
  Top 0.254: U1.17 15.89,11.54 16.26,11.18 16.89,11.18 17.27,11.56 v25.37,11.54 27.49,11.54 31.5,7.54 31.5,5.3 31.33,5.14 27.65,5.14 26.95,5.84 U$1.SCK
  Bottom 0.254: U$5.1 25.4,11.57 v25.37,11.54
D14  (via drill 0.35)  (2 unrouted)
  Top 0.203: U1.23 9.92,14.59 9.65,14.85 v9.65,17.9 v9.65,17.91 | v7.62,37.85 7.62,39.49 S1.3
  Top 0.254: R8.1 2.1,41.45 D1.1 1.91,39.62
  Bottom 0.203: v9.65,17.91 9.65,26.28 10.03,26.66 10.03,27.19 9.91,27.31 9.91,37.85 v7.62,37.85
D15  (via drill 0.35)  (1 unrouted)
  Top 0.203: U1.24 9.12,16.66 v8.89,16.89 | v14.61,24.64 14.61,28.08 16.63,30.11 16.63,33.28 15.72,34.19 15.72,34.8 15.72,39.34 v15.75,39.37 | v13.34,40.77 13.34,39.79 S2.4
  Top 0.254: S2.3 18.93,39.79 D2.1 19.31,41.66 R9.1
  Bottom 0.203: v8.89,16.89 10.04,16.89 12.06,18.91 12.06,18.92 14.48,21.34 14.48,21.72 14.61,21.84 14.61,22.48 14.48,22.61 14.48,24.51 v14.61,24.64 | v15.75,39.37 14.73,39.37 v13.34,40.77
D16  (via drill 0.35)
  Top 0.203: U1.25 7.63,18.93 7.75,19.05 9.89,19.05 10.85,20 10.85,20.07 10.85,25.58 11.43,26.16 11.68,26.16 12.7,27.18 12.7,28.19 12.45,28.45 12.32,28.45 11.05,29.72 11.05,34.42 12.32,35.69 12.32,35.82 12.42,35.92 12.42,40.15 11.7,40.87 11.43,40.87 10.19,40.87 9.53,41.53 9.53,44.83 v10.29,45.59 | v18.29,50.8 18.29,58.04 17.78,58.55 12.57,58.55 12.32,58.8 12.32,60.87 11.48,61.71 11.48,64.68 SW1.B
  Top 0.254: C13.1 R13.1 5.28,67.78 5.46,67.97 | 5.46,67.97 D6.1 | SW1.B 9.21,65.6 v8.64,65.02 | v6.37,65.15 6.37,67.8 6.35,67.82 5.61,67.82 5.46,67.97
  Bottom 0.203: v10.29,45.59 10.29,46.35 13.08,49.15 16.64,49.15 v18.29,50.8
  Bottom 0.254: v8.64,65.02 6.49,65.02 v6.37,65.15
D17  (via drill 0.35)  (1 unrouted)
  Top 0.203: U1.26 8.62,9.25 8.89,9.53 8.89,10.41 8.26,11.05 8.26,11.18 7.98,11.45 7.98,18.69 10.94,18.69 v11.43,19.18 | v13.84,22.1 13.84,27.82 15.72,29.7 15.72,32.74 v16,33.02 | v20.7,33.02 20.7,36.45 23.62,39.37 25.05,39.37 S3.4
  Top 0.254: S3.4 24.76,39.97 D3.1 24.89,41.42 24.89,42.8 24.44,43.25 R10.1
  Bottom 0.203: v11.43,19.18 11.43,19.68 v13.84,22.1 | v16,33.02 v20.7,33.02
D18  (via drill 0.35)  (1 unrouted)
  Top 0.203: U1.27 9.34,8.45 v9.53,8.64 | v10.29,15.11 10.29,16.13 12.19,18.03 12.19,24.81 S4.3
  Top 0.254: S4.4 12.24,32.01 D4.1 12.37,33.76 R11.1
  Bottom 0.203: v9.53,8.64 9.53,14.35 v10.29,15.11
D19  (via drill 0.35)  (1 unrouted)
  Top 0.203: U1.28 6.71,7.65 6.71,12.69 7.19,13.17 7.19,19.25 7.42,19.48 9.82,19.48 10.49,20.15 10.49,25.87 11,26.38 11,26.87 v11.56,27.43 | v25.91,28.45 25.91,29.24 25.59,29.56
  Top 0.254: S5.3 25.59,29.56 D5.1 27.2,27.75 R12.1
  Bottom 0.203: v11.56,27.43 24.89,27.43 v25.91,28.45
MISO2  (via drill 0.35)
  Top 0.254: v17.65,80.39 18.69,80.39 U2.11
  Bottom 0.254: v17.65,80.39 14.86,77.6 U$12.1 12.65,77.65 U$9.MISO
MOSI2  (via drill 0.35)
  Top 0.254: v16.26,80.26 16.51,80.26 17.4,79.38 17.65,79.38 18.03,79.76 18.19,79.76 U2.10
  Bottom 0.254: v16.26,80.26 14.99,79 U$13.1 12.62,78.92 U$9.MOSI
N$1
  Top 0.254: IC1.2 2.85,5.78 2.67,5.59 1.78,5.59 1.52,5.33 1.52,4.07 R1.2
N$2  (via drill 0.35)
  Top 0.254: v21.59,67.97 21.74,68.11 LED5.1 23.3,68.11 23.3,56.33 24.26,55.37 | LED7.1 8.07,68.45 v7.37,68.45 7.24,68.33 7.24,61.21 6.64,60.62 R28.1 | 24.26,55.37 24.89,54.74 26.97,54.74 LED3.1 | LED1.1 15.62,46.49 17.27,48.13 18.29,48.13 v22.73,52.58 | v23.62,54.74 23.63,54.74 24.26,55.37 | 4.29,54.84 LED9.1 4.31,54.73 4.95,55.37 7.25,55.37 10.08,52.53 10.08,48.91 11.34,47.66 12.99,47.66 v13.34,48.01
  Bottom 0.254: v21.59,67.97 21.49,67.97 20.83,67.31 16.13,67.31 15.49,67.94 7.87,67.94 v7.37,68.45 | v23.62,54.74 22.73,53.85 v22.73,52.58 18.16,48.01 v13.34,48.01
N$3  (via drill 0.35)
  Top 0.203: LED13.3 3.71,50.45 v3.3,50.04 | v7.62,22.23 6.73,22.23 5.46,20.95 4.06,20.95 2.92,19.81 C1.1 | IC1.8 1.58,11.24 1.65,11.18 5.33,11.18 5.59,10.92 5.59,7.09 IC1.4
  Top 0.406: C1.1 1.83,16.54 R17.2 1.84,12.66 IC1.8
  Bottom 0.203: v3.3,50.04 3.3,34.54 3.66,34.18 3.66,24.28 5.71,22.23 v7.62,22.23
N$4  (via drill 0.35)  (1 unrouted)
  Top 0.254: LED5.2 23.44,68.72 20.83,68.72 20.44,68.33 | 20.44,68.33 20.35,68.24 20.35,68.23 19.46,67.33 16.87,67.33 16.26,67.94 10.07,67.94 LED7.2 | 27.91,53.4 27.83,53.48 27.83,54.36 27.99,54.53 28.26,54.53 LED3.2 | 27.91,53.4 27.99,53.32 29.38,53.32 29.87,53.81 29.87,54.14 31.01,54.14 31.01,55.98 29.46,56.01 25.53,56.01 24.77,56.77 24.77,61.59 25.57,61.59 R29.1 | 24.77,61.47 24.77,63.75 25.15,64.14 v25.15,64.9 | v18.54,68.33 20.44,68.33 | 17.26,46.49 LED1.2 | 17.26,46.49 17.78,46.49 23.75,52.45 26.95,52.45 27.91,53.4 | LED9.2 6.04,54.48 7.56,54.48 9.68,52.37 9.68,48.74 11.68,46.74 12.57,46.74 v12.83,46.48 | v17.53,47.35 17.27,46.88 17.26,46.49
  Bottom 0.254: v18.54,68.33 19.18,68.96 23.24,68.96 23.88,68.33 23.88,65.02 25.02,65.02 v25.15,64.9 | v12.83,46.48 16.79,46.48 v17.53,47.35
N$5
  Top 0.254: Q1.1 1.46,57.96 R3.2 1.65,57.73 1.65,56.9 1.91,56.64 4.57,56.64 5.31,57.38 R2.1
N$6
  Top 0.254: R5.2 29.46,57.74 Q3.1 28.93,59.12 R4.1
N$7  (via drill 0.35)
  Top 0.254: LED7.4 9.8,67.37 9.53,67.37 9.37,67.53 9.37,68.42 9.53,68.58 10.56,68.58 10.76,68.38 15.61,68.38 16.48,69.25 | 16.48,69.25 | LED3.4 28.56,53.98 29.34,53.98 29.34,54.98 | 29.34,54.98 29.34,55.12 28.96,55.5 25.02,55.5 24.04,56.47 LED5.4 24.75,67.25 24.75,68.53 24.03,69.25 24.02,69.25 16.48,69.25 | v30.1,52.58 29.97,52.45 27.94,52.45 26.16,50.67 R30.1 22.99,50.67 17.95,45.64 LED1.4 17.14,45.6 17.14,44.7 13.08,44.7 9.27,48.51 9.27,52.2 7.59,53.88 LED9.4 | v30.1,54.99 29.35,54.99 29.34,54.98
  Bottom 0.254: v30.1,52.58 v30.1,54.99
N$8
  Top 0.254: R7.2 29.57,45.83 Q4.1 28.47,48.52 R6.1
N$9  (via drill 0.35)
  Top 0.203: R16.2 3.77,44.72 3.05,44 3.05,23.88 v4.06,22.86 | IC1.6 4.19,12.47 4.19,13.84 5.08,14.73 v5.08,18.29
  Bottom 0.203: v4.06,22.86 4.06,19.3 v5.08,18.29
N$10  (via drill 0.35)
  Top 0.203: R20.2 5.71,47.37 5.59,47.5 1.91,47.5 1.82,47.41 R18.2 1.82,45.68 v2.41,45.09 | v3.05,14.1 3.05,12.59 IC1.7
  Bottom 0.203: v2.41,45.09 2.41,34.92 3.3,34.04 3.3,14.35 v3.05,14.1
N$11
  Top 0.254: R16.1 3.77,48.6 4.7,49.53 7.37,49.53 7.62,49.78 7.62,50.42 LED13.4
N$12
  Top 0.254: R18.1 1.82,50.59 2.41,51.18 5.99,51.18 LED13.1
N$13  (via drill 0.35)
  Top 0.254: Q2.1 22.61,85.03 C9.1 22.67,86.67 v22.48,86.87 | v15.62,83.44 v15.63,83.44 U2.17
  Bottom 0.254: v22.48,86.87 19.05,86.87 v15.62,83.44
N$14
  Top 0.254: C3.2 12.15,12.87 12.32,12.7 U1.20
N$16
  Top 0.254: R20.1 7.2,48.35 8.64,49.78 8.64,51.18 8.51,51.31 7.61,51.31 LED13.2
N$17
  Top 0.254: J1.B5 7.78,27.08 8.89,28.19 8.89,28.83 9.4,29.34 9.4,31.24 8.89,31.75 8.89,34.42 10.29,35.81 10.29,38.16 9.95,38.5 9.67,38.5 R21.1
N$18
  Top 0.254: R22.2 4.83,36.83 3.81,35.81 3.81,31.04 4.75,30.1 6.71,30.1 J1.A5
N$19
  Top 0.254: U2.16 18.77,85.45 Q2.3 17.06,87.5 C8.1
N$20
  Top 0.254: C6.2 3.48,73.48 4.19,72.77 8.35,72.77 U2.42
N$21  (via drill 0.35)  (1 unrouted)
  Top 0.254: J1.VBUS1 7.53,31.28 8.26,32 8.26,33.27 v7.87,33.66 | v9.4,26.92 9.4,26.74 8.78,26.12
  Top 0.406: R17.1 3.74,18.53 6.17,20.95 9.14,20.95 9.16,20.97 9.16,25.77 8.96,25.97 8.93,25.97 8.78,26.12 8.5,26.4 6.83,26.4
  Bottom 0.254: v7.87,33.66 7.87,33.53 8.26,33.15 8.26,28.07 v9.4,26.92
N$22  (via drill 0.35)
  Top 0.406: U1.7 13.92,1.7 v14.1,1.52
  Bottom 0.406: v14.1,1.52 15.42,1.52 U$10.1
N$23
  Top 0.254: C7.1 1.16,72.76 1.78,72.14 12.06,72.14 12.83,72.9 12.83,74.42 14.1,76.07 14.1,77.47 15.95,77.47 U2.6
N$24  (via drill 0.35)
  Top 0.254: R23.1 20.86,80.24 20.57,80.52 19.3,80.52 18.29,81.53 18.29,81.58 | 18.29,81.58 U2.13 | v16.38,81.53 18.25,81.53 18.29,81.58
  Bottom 0.254: U$15.1 16.32,81.6 v16.38,81.53
N$25  (via drill 0.35)
  Top 0.406: U1.8 15.97,2.96 v16,2.92
  Bottom 0.406: v16,2.92 16.51,2.92 17.02,2.41 17.02,1.62 U$11.1
N$26
  Top 0.254: U2.3 15.22,74.82 17.04,73 19.47,73 20.26,73.79 23.62,73.79 23.62,76.45 23.37,76.71 22.73,76.71 22.73,77.78 R24.1
N$27
  Top 0.254: R25.1 20.79,74.89 19.3,73.41 17.75,73.41 U2.4
N$28
  Top 0.254: U$8.3 26.66,79.24 25.65,78.23 25.65,76.83 25.27,76.45 24.89,76.45 24.51,76.07 24.51,74.93 R25.2
N$29
  Top 0.254: U$8.2 26.37,81.24 25.78,80.64 25.78,79.5 25.4,79.12 24.51,79.12 24.38,78.99 24.38,77.91 R24.2
N$30
  Top 0.254: R26.2 21.17,2.79 R27.2 21.93,2.96 22.48,2.41 23.98,2.41 Q5.1
N$31  (via drill 0.35)
  Top 0.406: 24.35,1.53 Q5.3 | Q5.3 22.81,1.31 v22.73,1.39 | v18.16,2.92 C4.1 | Q5.3 31.02,1.31 IC2.1
  Bottom 0.406: v22.73,1.39 v22.73,1.4 21.21,2.92 v18.16,2.92
N$32
  Top 0.254: Q1.3 R28.2
N$33
  Top 0.254: Q3.3 27.79,61.86 R29.2
N$34
  Top 0.254: R30.2 30.48,50.67 Q4.3
PD9  (via drill 0.35)
  Top 0.254: v9.27,83.01 9.27,83.02 U2.29
  Bottom 0.254: U$9.CE 9.55,82.73 v9.27,83.01
PD10  (via drill 0.35)
  Top 0.254: U2.30 7.6,83.59 8.38,82.8 8.38,82.04 v8.51,81.92
  Bottom 0.254: v8.51,81.92 8.51,81.79 8.89,81.41 10.34,81.41 U$9.CSN
RESET  (via drill 0.35)
  Top 0.254: v22.86,10.74 15.44,10.74 14.99,10.29 14.99,9.4 v14.48,8.89 | v12.32,8.89 12.32,6.86 9.36,6.86 | 9.36,6.86 U1.29 7.62,6.86 | R19.2 6.58,2.87 v6.63,2.92 | v9.4,5.59 9.4,6.82 9.36,6.86
  Bottom 0.254: U$4.1 v22.86,10.74 | v14.48,8.89 v12.32,8.89 | v6.63,2.92 6.73,2.92 v9.4,5.59
SCK2  (via drill 0.35)
  Top 0.254: v14.73,80.39 14.86,80.39 16.76,78.49 17.27,78.49 17.75,78.97 17.85,78.97 U2.9
  Bottom 0.254: v14.73,80.39 14.52,80.18 U$14.1 12.69,80.19 U$9.SCK
V+  (via drill 0.35)
  Top 0.203: 6.16,55.78 6.15,55.79 6.15,57.99 6,58.14 4.69,58.14 4.12,58.71 4.12,60.92 4.76,61.56 5.99,61.56 6.14,61.71 6.14,62.92 3.81,65.25 R13.2 | LED7.3 8.55,65.83 8,65.29 8,61.98 8,60.07 8.76,59.31 8.76,54.54 8.71,54.48 | R8.2 6.82,43.34 v6.86,43.31 | v3.94,52.45 3.94,53.53 LED9.3 | 14.48,45.59 v13.97,45.59 | v22.61,45.59 22.61,43.8 22.68,43.73 | v27.56,43.18 27.56,34.54 30.1,32 30.1,30.35 30.35,30.1 30.35,27.43 30.23,27.3 29.35,27.3 | 29.35,27.3 R12.2 28.32,28.33 28.32,30.61 25.4,33.53 v23.5,33.53 | R11.2 14.2,34.57 v14.1,34.67 | CON1.2 18,22.95 v18.41,23.37 | v19.43,26.8 20.18,26.8 21.2,25.78 21.21,25.78 21.97,25.78 22.48,25.78 22.99,26.29 23.75,26.29 24.26,26.8 26.29,26.8 27.05,26.04 28.96,26.04 29.21,26.29 29.21,27.16 29.35,27.3
  Top 0.254: LED7.3 9.5,66.17 10.67,66.17 11.81,67.31 15.62,67.31 16,66.93 21.97,66.93 22.3,67.26 LED5.3 22.73,67.26 22.73,63.86 | LED3.3 26.93,53.85 22.73,53.85 22.73,53.98 | 22.73,63.86 22.73,62.85 | 22.73,61.84 22.73,62.85 | 22.73,61.84 22.73,53.98 | 22.73,53.98 17.91,49.15 17.27,49.15 | 17.27,49.15 15.62,47.5 14.99,47.5 14.48,46.99 14.48,45.59 15.57,45.59 LED1.3 | LED9.3 4.04,54.13 3.77,54.13 3.61,54.29 3.61,55.17 4.22,55.78 6.16,55.78 7.41,55.78 8.71,54.48 12.83,54.48 12.83,53.16 R14.2 14.79,53.02 17.14,50.67 17.14,49.28 17.27,49.15 | R15.2 28.75,63.42 28.19,62.87 v25.65,62.87 | v22.23,62.87 22.72,62.87 22.73,62.85 | v22.23,62.87 22.23,62.35 22.73,61.84 | v22.23,62.87 22.23,63.35 22.73,63.86 | U1.6 13.21,3.04 13.21,8.76 13.92,9.47 U1.18 13.97,11.59 v13.97,13.08 | R9.2 22.68,43.73 R10.2 | IC2.3 28.79,2.23 C5.2 25.45,2.23 v25.4,2.28 | 11.52,1.91 11.43,1.91 10.69,1.17
  Top 0.406: R19.1 10.69,1.17 12.47,1.17 v12.7,1.4 13.08,1.78 13.08,2.92 U1.6 | U1.4 11.52,1.91 10.83,1.22 | IC1.5 5.39,13.52 v5.71,13.84 | CON1.2 17.05,22 15.75,20.7 15.75,18.92 16.51,18.16 16.51,15.24 | 16.51,15.24 17.58,15.24 C2.2 | v13.97,13.08 13.97,15.24 14.1,15.37 16.38,15.37 16.51,15.24
  Bottom 0.203: v6.86,43.31 6.86,49.53 v3.94,52.45 | v13.97,45.59 v22.61,45.59 25.27,45.59 27.56,43.31 v27.56,43.18 | v14.1,34.67 22.35,34.67 v23.5,33.53 | v18.41,23.37 18.41,25.78 v19.43,26.8
  Bottom 0.254: v25.65,62.87 v22.23,62.87 | U$2.1 14.35,12.7 13.98,13.07 | v25.4,2.28 22.61,2.28 21.34,3.56 19.18,3.56 18.8,3.94 15.24,3.94 v12.7,1.4
  Bottom 0.406: v5.71,13.84 5.84,13.84 8,16 13.34,16 13.97,15.37 v13.97,13.08 13.98,13.07
VCC  (via drill 0.35)
  Top 0.254: U$8.1 25.74,83.74 24.45,82.45 24.45,80.26 R23.2 23.23,78.99 21.97,78.99 v20.32,77.34 | C10.1 20,75.76 19.43,76.33 19.3,76.33 | 19.3,76.33 18.54,76.33 18.41,76.2 18.36,76.2 U2.7 | IC3.3 0.93,81.63 C11.2 1.91,80.66 v1.91,79.63 | U2.14 18,82.42 v15.11,82.42 11.68,82.42 11.68,86.23 10.97,86.95 U2.24 | U2.34 4.98,79.34 v4.7,79.63 | U2.44 11.53,73.64 10.79,72.9 10.16,72.9 v10.03,73.03 | U2.2 v15.75,73.15 | v20.32,77.34 | v20.32,77.34 19.3,76.33
  Bottom 0.254: U$16.1 14.54,83 v15.11,82.42 18.29,82.42 20.7,80.01 20.7,77.72 v20.32,77.34 16.13,73.15 v15.75,73.15 10.16,73.15 v10.03,73.03 10.03,74.3 v4.7,79.63 v1.91,79.63
VCC/2  (via drill 0.35)
  Top 0.254: IC3.2 3.13,86.44 4.32,87.63 6.28,87.63 C12.2 8.09,87.56 v8.13,87.61
  Bottom 0.254: v8.13,87.61 8.13,87.54 U$9.3V3

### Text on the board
tNames: GREEN | RED | BLUE
bNames: v1.1 | v1.1

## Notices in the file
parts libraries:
SparkFun-IC-Microcontroller: Licensing: Creative Commons ShareAlike 4.0 International - https://creativecommons.org/licenses/by-sa/4.0
